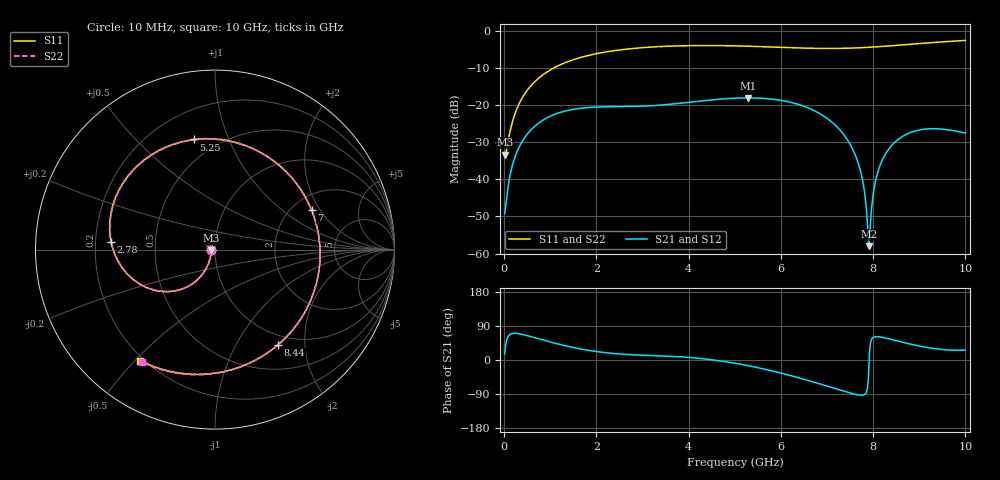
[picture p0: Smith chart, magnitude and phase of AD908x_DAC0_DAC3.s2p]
! Created Tue Jun 16 15:17:39 2020
# hz S ma R 50
! 2 Port Network Data from SP1.SP block
! freq  magS11  angS11  magS21  angS21  magS12  angS12  magS22  angS22
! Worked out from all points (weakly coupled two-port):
!   1000 points, 10 MHz to 10 GHz, reference 50 ohm
!   highest |S21| = -18.04 dB at 5.28 GHz (marker M1); lowest = -58.0 dB at 7.91 GHz (marker M2)
!   lowest |S11| = -33.3 dB at 20 MHz (marker M3), VSWR 1.04, Z = 47.9 - j0.298 ohm
!   |S11| at or under -10 dB: start of sweep to 1.072 GHz
!   |S22| runs from -33.4 to -2.5 dB; largest |S21 - S12| = 0
!   S11 on the Smith chart (normalised r, x): 10 MHz: 0.95, -0.00; 2.78 GHz: 0.27, +0.03; 5.25 GHz: 0.38, +0.76; 7 GHz: 2.53, +1.68; 8.44 GHz: 0.85, -1.51; 10 GHz: 0.19, -0.52
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1e7  0.02302 -179.0  0.003425 15.8  0.003425 15.8  0.02308 -179.4
2e7  0.02162 -171.7  0.003742 27.1  0.003742 27.1  0.02156 -172.6
2e8  0.06582 -117.3  0.01718 70.3  0.01718 70.3  0.06523 -117.5
4.9e8  0.1557 -117.1  0.03988 64.6  0.03988 64.6  0.1545 -117.1
9.8e8  0.2932 -130.7  0.07004 48.2  0.07004 48.2  0.2911 -130.6
1.68e9  0.4435 -152.2  0.09116 28.6  0.09116 28.6  0.4408 -152.0
2.78e9  0.5801 176.0  0.09605 13.9  0.09605 13.9  0.5775 176.3
3.34e9  0.6151 160.2  0.09971 11.3  0.09971 11.3  0.6126 160.5
5.01e9  0.63 109.3  0.1243 -8.7  0.1243 -8.7  0.6281 109.6
5.25e9  0.6245 100.8  0.1253 -14.0  0.1253 -14.0  0.6228 101.1
5.28e9  0.6237 99.7  0.1253 -14.7  0.1253 -14.7  0.6221 100.0
6.67e9  0.5847 39.5  0.08751 -56.8  0.08751 -56.8  0.5841 39.9
7e9  0.5814 22.3  0.06655 -68.8  0.06655 -68.8  0.581 22.6
7.37e9  0.5845 2.0  0.03959 -82.4  0.03959 -82.4  0.5842 2.3
7.63e9  0.5915 -12.6  0.02002 -90.9  0.02002 -90.9  0.5912 -12.2
7.77e9  0.5969 -20.4  0.009799 -92.7  0.009799 -92.7  0.5967 -20.0
7.91e9  0.6034 -28.1  0.001257 -11.0  0.001257 -11.0  0.6032 -27.7
8.08e9  0.6126 -37.4  0.01122 61.7  0.01122 61.7  0.6125 -37.0
8.34e9  0.629 -51.3  0.02568 55.9  0.02568 55.9  0.6289 -50.8
8.44e9  0.6359 -56.4  0.03034 52.8  0.03034 52.8  0.6359 -55.9
9.07e9  0.6824 -86.6  0.0471 35.3  0.0471 35.3  0.6832 -85.9
1e10  0.7456 -124.0  0.04212 26.2  0.04212 26.2  0.748 -123.1
